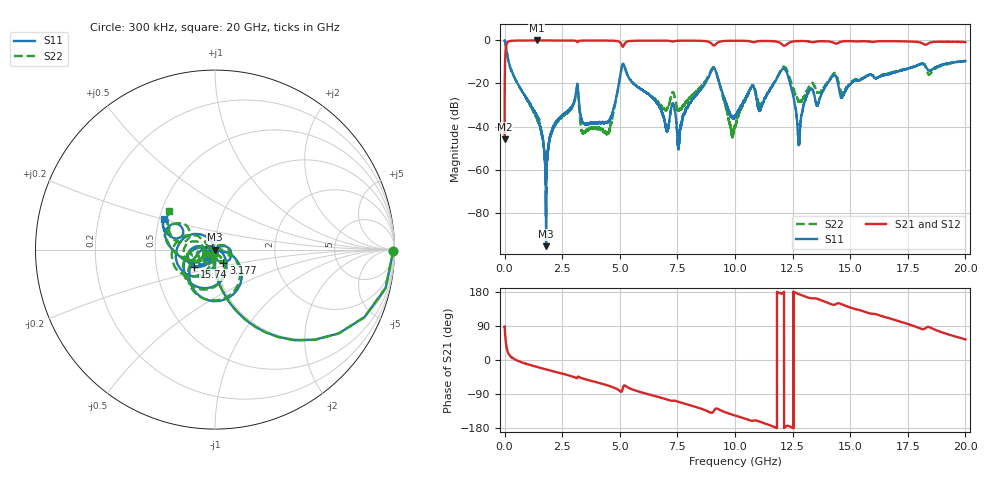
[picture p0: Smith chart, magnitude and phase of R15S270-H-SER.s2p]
!{R15S270}
!Johanson Technology Inc.
!www.johansontechnology.com
!Test Board Conditions:
!Substrate Type  RO4350B
!Substrate Thickness  20 mil
!Substrate Dk  3.66
!TL Type: GCPW
!TL Trace Width  34 mil
!TL Gap  10 mil
!Electrode orientation  Horizontal
!DUT TOPOLOGY	SERIES
!Mounting Pad LxW  26x52 mil
! Created Sat Feb  6 14:24:24 2021
# hz S ma R 50
! 2 Port Network Data from SP1.SP block
! freq  magS11  angS11  magS21  angS21  magS12  angS12  magS22  angS22
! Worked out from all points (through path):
!   20001 points, 300 kHz to 20 GHz, reference 50 ohm
!   highest |S21| = -0.01 dB at 1.388 GHz (marker M1); lowest = -45.9 dB at 300 kHz (marker M2)
!   group delay of S21, straight-line fit = 42.6 ps
!   lowest |S11| = -95.6 dB at 1.8 GHz (marker M3), VSWR 1.00, Z = 50 + j2.66e-05 ohm
!   |S11| at or under -10 dB: 176.4 MHz to 19.59 GHz (19.41 GHz wide, 196 % of centre); 19.59345 GHz to 19.5972 GHz (3.755 MHz wide, 0.0192 % of centre); 19.59741 GHz to 19.60213 GHz (4.721 MHz wide, 0.0241 % of centre)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
!   |S22| runs from -67.3 to 0.0 dB; largest |S21 - S12| = 0.014
!   S11 on the Smith chart (normalised r, x): 300 kHz: open; 3.177 GHz: 1.08, -0.16; 15.74 GHz: 0.78, -0.15; 20 GHz: 0.53, +0.20
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300000  0.9931 -0.5  0.005046 88.3  0.005022 89.2  0.9938 -0.4
1.483e8  0.3694 -70.2  0.9265 19.6  0.9274 19.5  0.371 -70.1
1.3883e9  0.01827 -105.9  0.9991 -18.1  0.9978 -18.1  0.01632 -110.5
1.8003e9  1.664e-05 0.9  0.9977 -24.8  0.9983 -24.8  0.0005113 4.8
2.1433e9  0.01017 52.1  0.9974 -30.3  0.9971 -30.3  0.009973 62.2
3.1773e9  0.08634 -57.7  0.9205 -44.2  0.9208 -44.1  0.0729 -65.9
3.3343e9  0.01497 -74.5  0.9927 -47.6  0.9929 -47.7  0.008756 -169.3
4.4913e9  0.013 -49.5  0.9923 -67.4  0.9927 -67.5  0.007533 68.6
5.1523e9  0.287 -94.8  0.7289 -70.7  0.7288 -70.7  0.2828 -98.5
6.6673e9  0.03263 148.2  0.9907 -97.5  0.9895 -97.5  0.03686 -150.8
7.0463e9  0.007796 65.8  0.987 -104.2  0.9859 -104.1  0.02572 -103.0
7.3233e9  0.03289 -115.0  0.9464 -107.2  0.948 -107.2  0.06135 -115.9
7.5723e9  0.004921 68.4  0.9853 -110.9  0.9859 -110.8  0.02341 -93.5
9.0723e9  0.2306 -119.7  0.7644 -135.2  0.7664 -135.3  0.2386 -121.5
1.00003e10  0.0172 -121.7  0.9836 -146.4  0.9831 -146.5  0.01029 -82.5
1.07143e10  0.08292 -113.8  0.9356 -160.4  0.9362 -160.4  0.08309 -108.4
1.21193e10  0.2243 -164.5  0.7588 179.3  0.7619 179.2  0.2445 -164.3
1.27813e10  0.004972 -164.3  0.9683 173.7  0.9668 173.7  0.0369 170.7
1.33343e10  0.07401 -151.7  0.9143 162.7  0.9147 162.6  0.1029 -162.1
1.57383e10  0.151 -140.6  0.9546 125.0  0.9545 125.2  0.1525 -156.9
1.66673e10  0.1646 -156.4  0.9611 110.6  0.9515 110.6  0.174 -165.4
2e10  0.3312 149.2  0.9167 54.4  0.9135 54.2  0.3325 139.8
